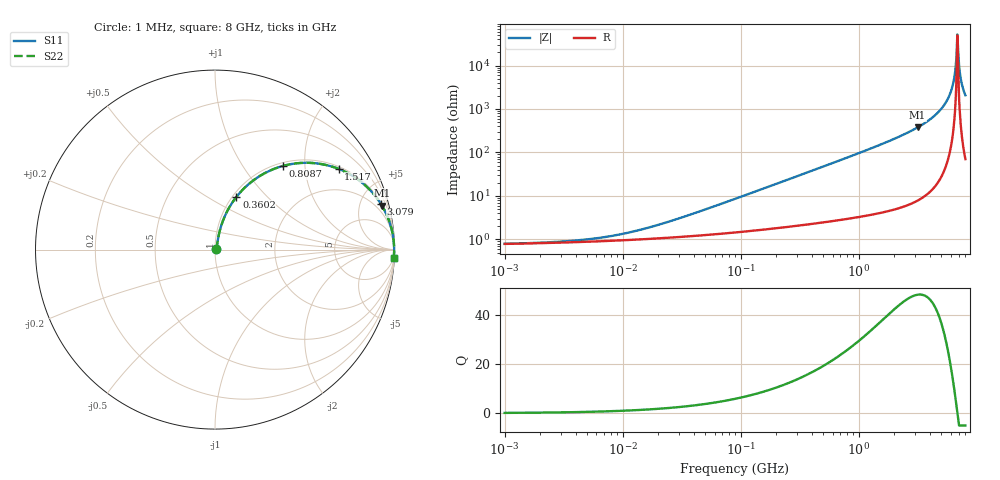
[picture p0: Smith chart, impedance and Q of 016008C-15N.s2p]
# MHz S MA R 50
!Freq  MagS11  AngS11  MagS21  AngS21  MagS12  AngS12  MagS22  AngS22
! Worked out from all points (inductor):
!   801 points, 1 MHz to 8 GHz, reference 50 ohm
!   read as one part in series: L = 15 nH near 38.08 MHz
!   highest Q = 48.3 at 3.149 GHz (marker M1), where L = 19 nH
!   self-resonance near 6.836 GHz
!   S11 on the Smith chart (normalised r, x): 1 MHz: 1.02, +0.00; 360.2 MHz: 1.04, +0.68; 808.7 MHz: 1.06, +1.55; 1.517 GHz: 1.08, +3.01; 3.079 GHz: 1.15, +7.27; 8 GHz: 2, -41
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1  0.007869 6.8  0.9922 -0.1  0.9922 -0.1  0.007869 6.8
4.505755  0.009637 25.7  0.9913 -0.2  0.9913 -0.2  0.009637 25.7
9.457416  0.01289 42.7  0.9906 -0.5  0.9906 -0.5  0.01289 42.7
20.07503  0.02144 59.7  0.9894 -1.1  0.9894 -1.1  0.02144 59.7
90.45318  0.08495 75.6  0.9823 -4.8  0.9823 -4.8  0.08495 75.6
360.1836  0.3167 67.9  0.9284 -18.4  0.9284 -18.4  0.3167 67.9
403.007  0.3498 66.1  0.9162 -20.4  0.9162 -20.4  0.3498 66.1
808.7272  0.6008 50.9  0.7766 -36.9  0.7766 -36.9  0.6008 50.9
1517.114  0.8226 33.1  0.5469 -55.3  0.5469 -55.3  0.8226 33.1
1795.566  0.8671 28.5  0.4771 -60.1  0.4771 -60.1  0.8671 28.5
3078.837  0.9591 15.3  0.2637 -73.5  0.2637 -73.5  0.9591 15.3
3148.795  0.9615 14.8  0.2555 -74.0  0.2555 -74.0  0.9615 14.8
4410.728  0.9871 8.0  0.139 -80.7  0.139 -80.7  0.9871 8.0
5521.887  0.9954 3.8  0.06696 -84.2  0.06696 -84.2  0.9954 3.8
6178.402  0.9974 1.8  0.03194 -84.5  0.03194 -84.5  0.9974 1.8
6390.175  0.9978 1.2  0.02152 -83.5  0.02152 -83.5  0.9978 1.2
6609.207  0.998 0.6  0.01117 -79.6  0.01117 -79.6  0.998 0.6
6835.746  0.9982 0.0  0.001929 -17.5  0.001929 -17.5  0.9982 0.0
7070.05  0.9982 -0.6  0.01 79.2  0.01 79.2  0.9982 -0.6
7312.386  0.9981 -1.2  0.02035 83.9  0.02035 83.9  0.9981 -1.2
7563.027  0.9978 -1.8  0.03077 85.1  0.03077 85.1  0.9978 -1.8
8000  0.9972 -2.8  0.04823 85.3  0.04823 85.3  0.9972 -2.8
